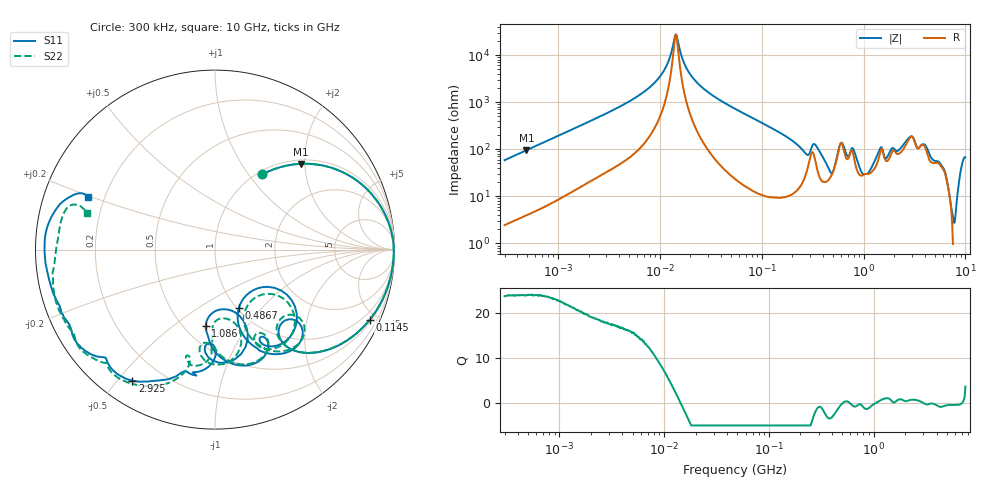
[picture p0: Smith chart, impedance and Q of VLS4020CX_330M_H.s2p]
! S-Parameter Data Generated by TDK Corporation
! Copyright(C) 2024 TDK Corporation.
! All Rights Reserved.
! TDK P/N: VLS4020CX-330M-H (SMD / SMT Inductor (Coil))
! Property: L=33uH at 1MHz
! Size(LxWxT): 4x4x2mm
! Model Type: s2p (Touchstone File Format Version 1.0)
! Frequency: DC=Yes Start=0.3MHz Stop=10000MHz 802points Log-sweep
! Model Generated on May 28, 2024
! Terms and conditions regarding TDK Simulation Models:
! 1)This simulation model is being provided solely for informational
!  purposes. Please refer to the specifications of the products in
!  terms of detailed characteristics of such products.
! 2)In no event shall TDK Corporation of any of its subsidiaries be
!  liable for any loss or damage arising, directly or indirectly,
!  from any information contained in this simulation model, including,
!  but not limited to loss or damages arising from any inaccuracies,
!  omissions or errors in connection with such information.
! 3)Any and all copyrights on this simulation model are owned by
!  TDK Corporation.  Duplication or redistribution of this simulation
!  model without prior written permission from TDK Corporation
!  is prohibited.
! 4)This simulation model is subject to any modification or change
!  without any prior notice.
! 5)Neither TDK Corporation nor any of its subsidiaries shall make any
!  warranty, express or implied, including but not limited to the
!  correctness, implied warranties of merchantability and fitness for
!  a particular purpose with respect to this simulation models.
! 6)The use of this simulation model shall be deemed to have consented
!  to the terms and conditions hereof.
! Port Assignments:
!  1 ---@@@--- 2
! Applicable Conditions:
!  Temperature = 25 degC
!  DC Bias Current = 0 A
!  Small Signal Operation
# Hz S MA R 50
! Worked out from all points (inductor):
!   801 points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, 300 kHz to 10 GHz, reference 50 ohm
!   read as one part in series: L = 30.9 uH near 318.3 kHz
!   highest Q = 24.1 at 491.6 kHz (marker M1), where L = 30.8 uH
!   self-resonance near 14.38 MHz
!   S11 on the Smith chart (normalised r, x): 300 kHz: 1.05, +1.17; 114.5 MHz: 0.61, -4.53; 486.7 MHz: 1.02, -0.76; 1.086 GHz: 0.63, -0.66; 2.925 GHz: 0.10, -0.55; 10 GHz: 0.14, +0.19
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300000  0.4949 57.8  0.8483 -29.8  0.8483 -29.8  0.495 57.8
491566  0.6749 45.1  0.7099 -42.6  0.7101 -42.5  0.6751 45.1
1713600  0.9428 16.7  0.2893 -70.4  0.2894 -70.5  0.9428 16.7
9671944  0.9955 1.2  0.03159 -81.5  0.0316 -81.5  0.9955 1.2
1.43789e7  0.9963 -0.9  0.003645 -2.6  0.003651 -2.6  0.9964 -0.9
2.063197e7  0.996 -2.9  0.02849 79.8  0.02852 79.9  0.996 -2.9
5.477226e7  0.9863 -11.3  0.1359 76.9  0.136 76.9  0.9863 -11.3
1.145169e8  0.9462 -24.5  0.2959 63.8  0.2959 63.8  0.946 -24.4
2.195581e8  0.7874 -47.0  0.5486 37.8  0.5487 37.8  0.7857 -47.0
2.725454e8  0.6065 -53.6  0.6287 17.6  0.6288 17.6  0.5952 -54.0
3.126428e8  0.6275 -41.2  0.4717 7.6  0.4717 7.6  0.6089 -39.0
3.7738e8  0.6589 -61.8  0.6141 16.5  0.6142 16.5  0.6612 -59.1
4.866838e8  0.352 -67.9  0.7305 -12.6  0.7306 -12.6  0.3811 -63.9
5.99416e8  0.6019 -40.8  0.3926 -26.2  0.3927 -26.2  0.6197 -44.6
8.299813e8  0.664 -76.8  0.5032 -12.0  0.5033 -12.0  0.661 -75.4
1.085776e9  0.4285 -97.0  0.663 -41.0  0.6632 -41.0  0.4437 -91.7
1.403063e9  0.474 -68.1  0.4933 -81.4  0.4935 -81.4  0.5217 -73.6
1.767019e9  0.5407 -90.3  0.4404 -90.5  0.441 -90.5  0.5449 -92.3
2.924554e9  0.8628 -122.3  0.1139 -115.6  0.1138 -115.8  0.8753 -121.0
5.849356e9  0.9213 -159.5  0.08705 -109.2  0.08688 -109.3  0.9261 -153.7
7.222042e9  0.947 -175.2  0.08238 -118.1  0.08247 -118.0  0.9146 -171.8
1e10  0.7669 157.6  0.05285 -130.1  0.0528 -130.1  0.742 164.1
